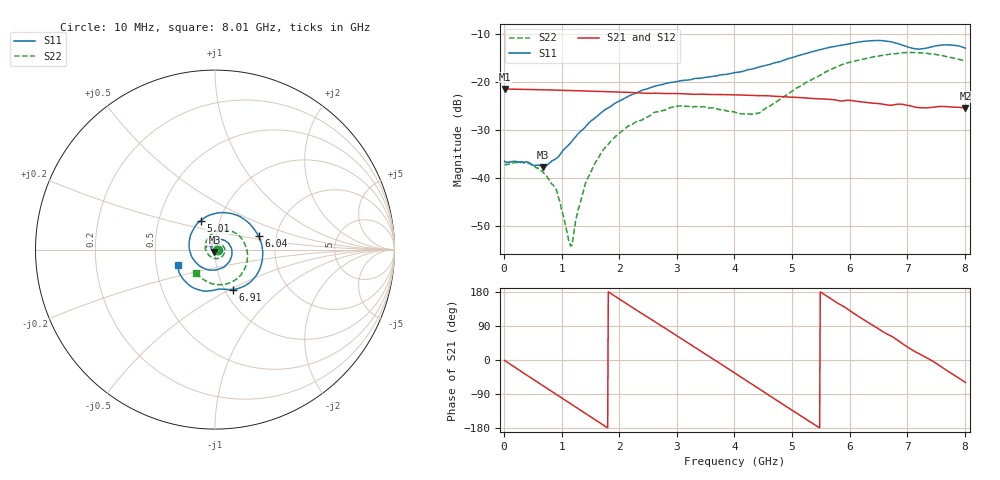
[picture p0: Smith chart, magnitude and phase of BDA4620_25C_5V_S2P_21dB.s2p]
!Agilent Technologies,E5071B,MY42404982,A.09.10
!Date: Wed May 06 09:02:51 2026
!Data & Calibration Information:
!Freq	S11:SOLT2(ON)	S21:SOLT2(ON)	S12:SOLT2(ON)	S22:SOLT2(ON)
# Hz S RI R 50
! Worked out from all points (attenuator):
!   801 points, 10 MHz to 8.01 GHz, reference 50 ohm
!   highest |S21| = -21.41 dB at 10 MHz (marker M1); lowest = -25.5 dB at 8.01 GHz (marker M2)
!   lowest |S11| = -37.8 dB at 680 MHz (marker M3), VSWR 1.03, Z = 49.7 - j1.25 ohm
!   |S11| at or under -10 dB: start of sweep to end of sweep
!   |S22| runs from -54.2 to -13.8 dB; largest |S21 - S12| = 0.00036
!   S11 on the Smith chart (normalised r, x): 10 MHz: 1.03, -0.00; 5.01 GHz: 0.81, +0.27; 6.04 GHz: 1.61, +0.26; 6.91 GHz: 1.10, -0.52; 8.01 GHz: 0.65, -0.12
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1e7  0.0149 -0.00102  0.085 -0.0018  0.0852 -0.00181  0.0137 -0.000478
4.2e8  0.00835 -0.0119  0.0617 -0.0565  0.0618 -0.0567  0.0133 -0.00481
6.8e8  -0.00292 -0.0126  0.0306 -0.0773  0.0306 -0.0774  0.00917 -0.00683
9.2e8  -0.0148 -0.00648  -0.00334 -0.0823  -0.00338 -0.0824  0.00352 -0.00619
1.15e9  -0.0219 0.0072  -0.0347 -0.0739  -0.0349 -0.0741  -0.00158 -0.00122
1.19e9  -0.0224 0.0103  -0.0397 -0.0712  -0.0398 -0.0713  -0.0022 6.7e-05
1.35e9  -0.0219 0.0225  -0.0573 -0.0573  -0.0573 -0.0573  -0.00375 0.00508
1.53e9  -0.0156 0.0371  -0.0713 -0.0369  -0.0715 -0.0369  -0.0035 0.0118
1.77e9  0.00232 0.0521  -0.0794 -0.0052  -0.0795 -0.00512  0.000927 0.0212
2.15e9  0.0451 0.0545  -0.0651 0.0434  -0.0652 0.0435  0.0177 0.0298
2.68e9  0.0926 0.00235  -0.00677 0.076  -0.00669 0.0761  0.0454 0.0191
3.08e9  0.0823 -0.0631  0.0422 0.0629  0.0425 0.0629  0.0557 -0.00821
4.01e9  -0.0892 -0.0884  0.0604 -0.0421  0.0604 -0.0423  -0.0117 -0.0473
4.42e9  -0.143 0.00336  0.0186 -0.0698  0.0185 -0.0699  -0.0459 -0.0125
5.01e9  -0.0803 0.1619  -0.0478 -0.0507  -0.048 -0.0506  -0.0308 0.0751
5.35e9  0.0278 0.2058  -0.0657 -0.0156  -0.0658 -0.0156  0.0234 0.1038
6.04e9  0.2425 0.0763  -0.0379 0.0517  -0.038 0.0519  0.1544 0.0541
6.36e9  0.2626 -0.0617  -0.00575 0.0604  -0.00576 0.0605  0.1799 -0.014
6.68e9  0.1877 -0.1882  0.0233 0.0524  0.0235 0.0526  0.1714 -0.0918
6.91e9  0.1003 -0.2224  0.0424 0.0406  0.0425 0.0407  0.1432 -0.1425
7.57e9  -0.0902 -0.2246  0.0537 -0.015  0.0538 -0.015  -0.0173 -0.1897
8.01e9  -0.2087 -0.0856  0.0272 -0.0459  0.0274 -0.046  -0.1053 -0.1279
